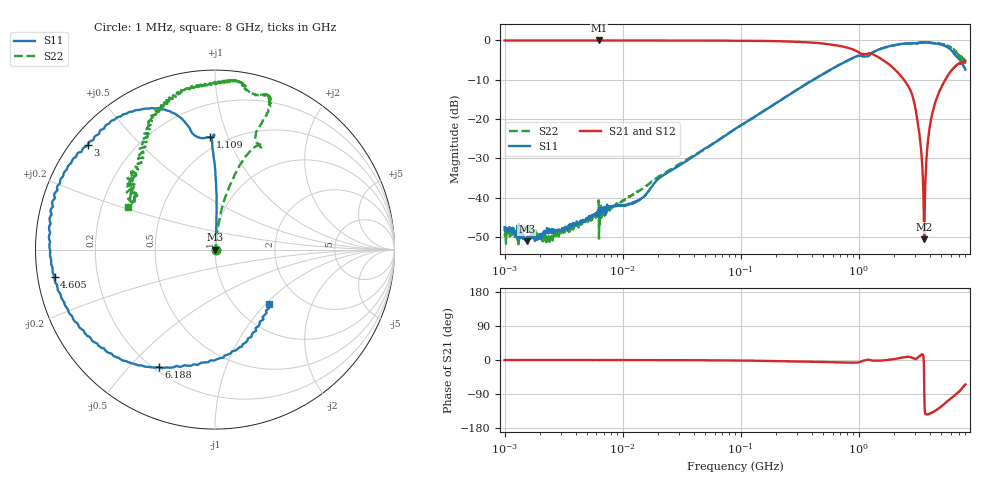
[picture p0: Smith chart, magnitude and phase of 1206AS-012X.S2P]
!s-Parameter Generated by FASTRON Sdn. Bhd.
!FASTRON P/N : 1206AS-012X
!Keysight Technologies: E5071C_MY46733604_B.14.02
!Date: Wed Nov 15 09:38:44 2023
!Version  :Rev00  Wed Nov 15 09:38:44 2023
!Data & Calibration Information:
!Freq  S11:SOLT2(ON)  S21:SOLT2(ON)  S12:SOLT2(ON)  S22:SOLT2(ON)
!PortZ  Port1:50+j0  Port2:50+j0
!When reading reference impedance value at option line is always used.
! Remarks : This data is being provided solely for informational purposes.
# Hz S dB R 50
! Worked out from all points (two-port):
!   1601 points, 1 MHz to 8 GHz, reference 50 ohm
!   highest |S21| = -0.02 dB at 6.301 MHz (marker M1); lowest = -50.6 dB at 3.589 GHz (marker M2)
!   |S21| within 3 dB of the highest: start of sweep to 995.5 MHz
!   lowest |S11| = -51.1 dB at 1.541 MHz (marker M3), VSWR 1.01, Z = 50.3 - j0.064 ohm
!   |S11| at or under -10 dB: start of sweep to 413.6 MHz
!   |S22| runs from -52.3 to -0.5 dB; largest |S21 - S12| = 0.006
!   S11 on the Smith chart (normalised r, x): 1 MHz: 1.01, -0.00; 1.109 GHz: 0.42, +0.87; 3 GHz: 0.05, +0.36; 4.605 GHz: 0.05, -0.08; 6.188 GHz: 0.22, -0.61; 8 GHz: 1.41, -1.04
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1000000  -47.53 -18.7  -0.03 -0.2  -0.04 -0.1  -49.39 -21.6
1541011  -51.07 -13.2  -0.02 -0.2  -0.03 -0.1  -47.79 -23.7
2211112  -49.13 20.9  -0.03 -0.1  -0.03 -0.1  -50.75 44.3
4479405  -45.95 45.0  -0.03 -0.1  -0.04 -0.1  -46.77 51.2
6301378  -42.54 37.1  -0.02 -0.3  -0.01 -0.1  -50.40 30.3
1.345746e7  -40.84 78.0  -0.03 -0.3  -0.05 -0.3  -38.51 64.6
2.00676e7  -35.20 76.6  -0.04 -0.4  -0.05 -0.3  -34.73 75.7
8.994653e7  -22.49 85.4  -0.08 -1.3  -0.09 -1.3  -22.59 82.9
4.006501e8  -10.25 88.4  -0.56 -4.5  -0.57 -4.5  -10.26 78.6
1.108954e9  -4.07 92.5  -3.45 -1.3  -3.46 -1.4  -4.07 66.4
1.7949e9  -1.54 111.0  -6.03 0.4  -6.05 0.2  -1.56 69.1
2.604275e9  -0.73 129.5  -11.46 8.6  -11.50 8.4  -0.82 71.8
3.000426e9  -0.76 140.7  -16.85 3.3  -16.88 3.3  -0.96 77.2
3.26428e9  -0.56 148.3  -23.84 9.5  -23.85 9.5  -0.65 79.4
3.466968e9  -0.53 153.9  -33.05 14.5  -33.08 14.5  -0.51 81.0
3.588581e9  -0.53 157.1  -50.56 -86.1  -50.53 -86.4  -0.46 82.9
3.689925e9  -0.51 160.0  -33.86 -142.9  -33.84 -142.9  -0.46 83.8
3.831807e9  -0.55 164.6  -26.31 -143.2  -26.31 -143.4  -0.55 86.5
3.993958e9  -0.55 169.3  -22.02 -141.4  -22.02 -141.5  -0.57 87.2
4.604562e9  -0.85 -170.3  -14.52 -131.0  -14.49 -131.1  -0.74 96.0
6.187922e9  -2.79 -115.6  -7.38 -98.6  -7.36 -98.9  -2.12 118.2
8e9  -7.40 -45.3  -5.18 -64.5  -5.17 -65.1  -5.35 154.1
